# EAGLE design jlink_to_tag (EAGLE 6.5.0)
AUTHOR: Noah Klugman / Brad Campbell; REV: B; TITLE: JLink to Tag Connect
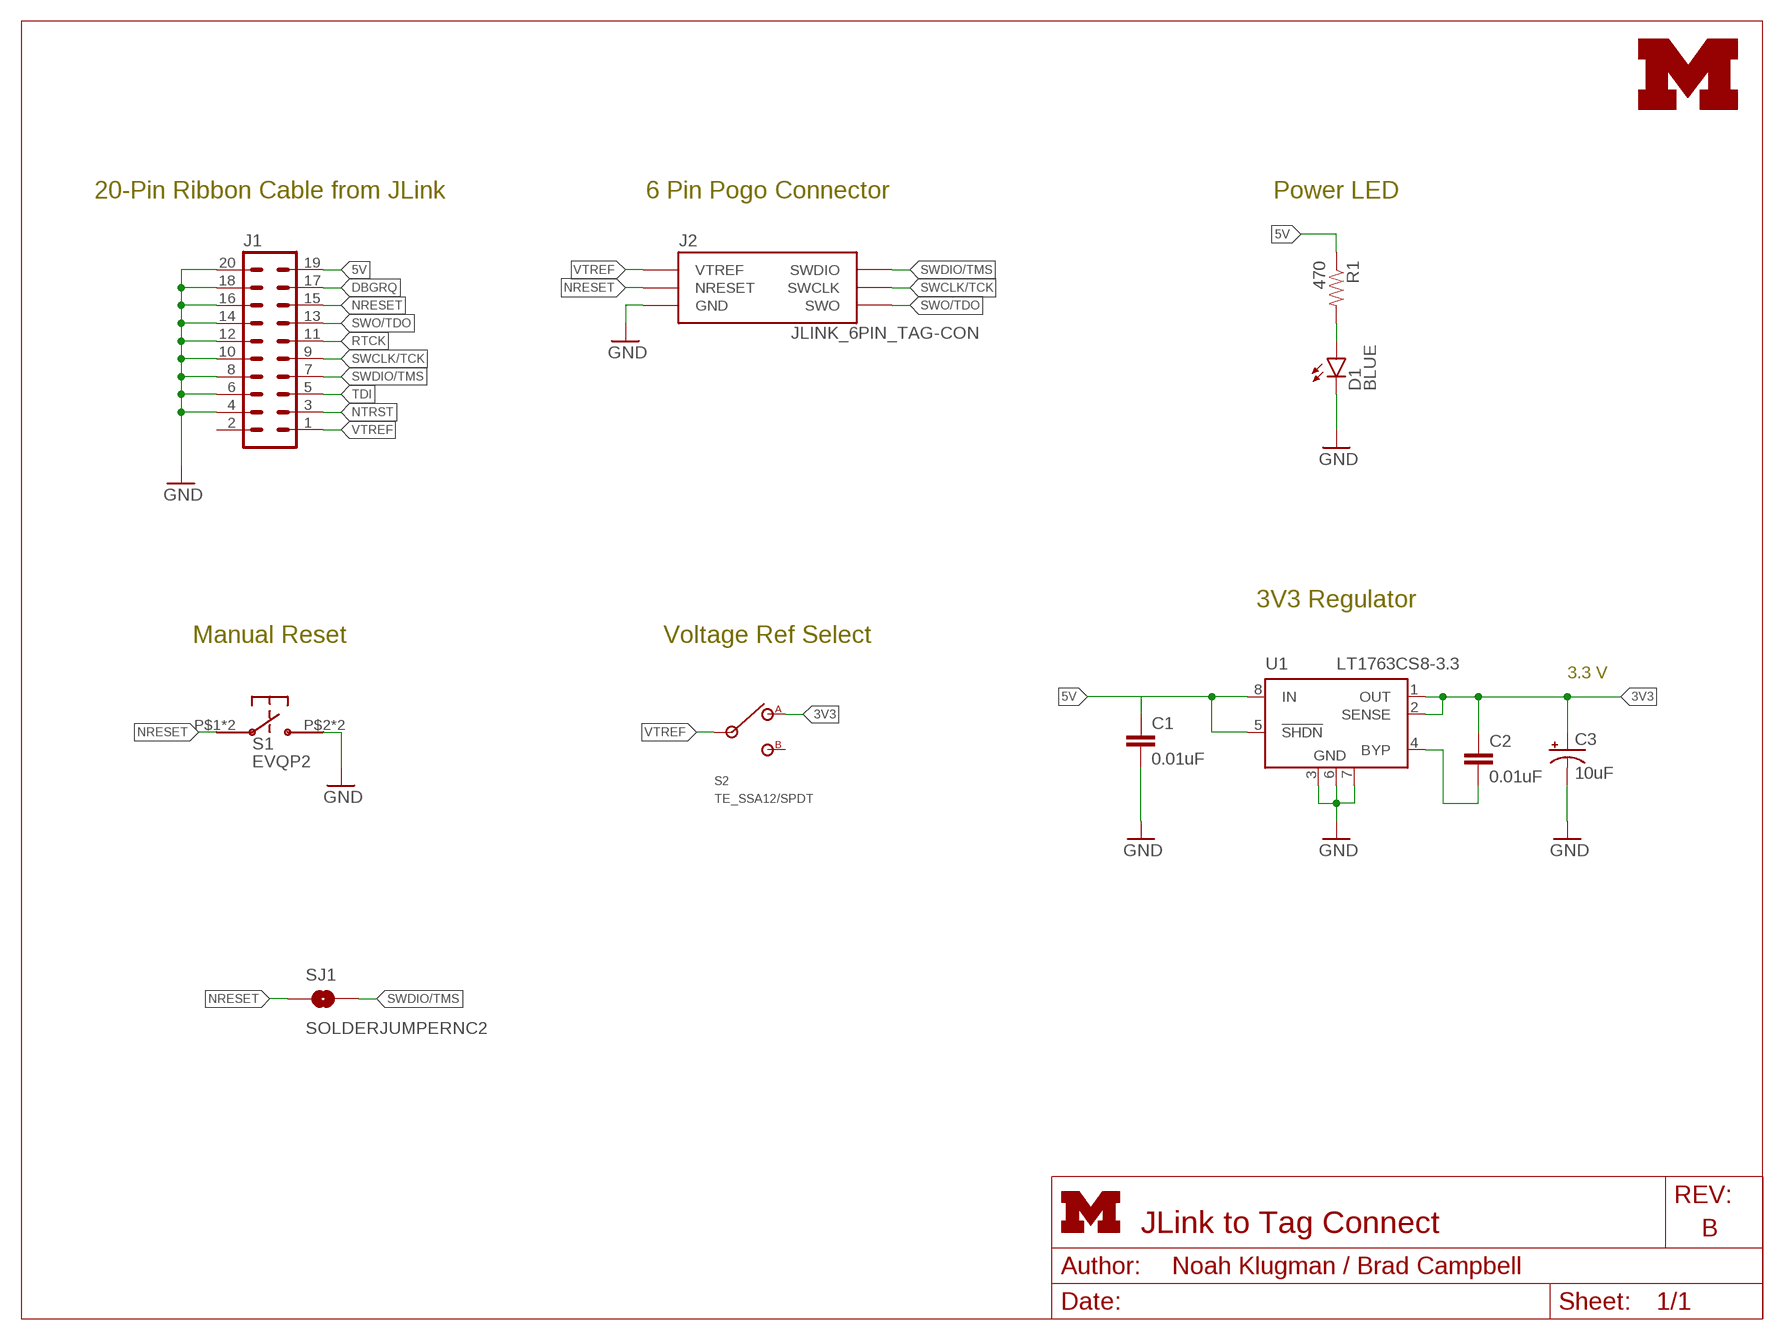
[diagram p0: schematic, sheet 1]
FRAME1 (LETTER_L): HEIGHT: 8.5in; WIDTH: 11in

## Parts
C1  0.01uF  C-EUC0603  [C0603]
C2  0.01uF  C-EUC0603  [C0603]
C3  10uF  CAP_POL1206  [EIA3216]
D1  BLUE  LED-BLUE0603  [LED-0603]
J1  ML20  [ML20]
J2  JLINK_6PIN_TAG-CON  [2X3_MALE_SHROUDED_0.100]
LOGO1  UMICH_SOLID_SMALL+  [UMICH_SOLID_100MIL]
R1  470  RESISTOR0603-RES  [0603-RES]
S1  EVQP2  [EVQP2]
S2  TE_SSA12/SPDT  [TE_SSA12/SPDT]
SJ1  SOLDERJUMPERNC2  [SJ_2S-NOTRACE]
U1  LT1763CS8-3.3  [SOIC8]

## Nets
3V3: C2.1 C3.A(+) S2.1(A) U1.1(OUT) U1.2(SENSE)
5V: C1.1 J1.19 R1.1 U1.5(!SHDN) U1.8(IN)
DBGRQ: J1.17
GND: C1.2 C3.C(-) D1.C J1.4 J1.6 J1.8 J1.10 J1.12 J1.14 J1.16 J1.18 J1.20 J2.5(GND) S1.P$2 S1.P$4 U1.3(GND) U1.6(GND) U1.7(GND)
N$3: D1.A R1.2
N$4: C2.2 U1.4(BYP)
NRESET: J1.15 J2.3(NRESET) S1.P$1 S1.P$3 SJ1.1
NTRST: J1.3
RTCK: J1.11
SWCLK/TCK: J1.9 J2.4(SWCLK)
SWDIO/TMS: J1.7 J2.2(SWDIO) SJ1.2
SWO/TDO: J1.13 J2.6(SWO)
TDI: J1.5
VTREF: J1.1 J2.1(VTREF) S2.IN
Unconnected: J1.2 S2.2(B)

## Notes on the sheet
- 20-Pin Ribbon Cable from JLink | 6 Pin Pogo Connector | Power LED
- 3V3 Regulator
- Manual Reset | Voltage Ref Select
- 3.3 V

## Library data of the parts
C1 C2 = resistor:C-EU: CAPACITOR, European symbol; DIGIKEY: 490-1512-1-ND
C3 = SparkFun-Passives:CAP_POL: Capacitor Polarized; DIGIKEY: 399-3684-1-ND
D1 = SparkFun-LED:LED-BLUE: Blue LEDs for production use; PROD_ID: DIO-08575
J1 = con-ml:ML20: HARTING; DIGIKEY: S9172-ND; OC_FARNELL: unknown; OC_NEWARK: unknown
J2 = headers:JLINK_6PIN_TAG-CON: This is a 6-pin Tag Connect header with the J-Link.; DIGIKEY: 3M15451-ND
LOGO1 = logos:UMICH_SOLID
R1 = SparkFun-Passives:RESISTOR: Resistor
S1 = switches:EVQP2: SWITCH TACTILE SPST-NO 0.02A 15V; DIGIKEY: P11084SCT-ND
S2 = switches:TE_SSA12/SPDT: SWITCH SLIDE SPDT 2POS SSA SER; DIGIKEY: 450-1602-ND
SJ1 = SparkFun-Passives:SOLDERJUMPER: Solder Jumper
U1 = linear-technology:LT1763CS8: 500mA, Low Noise, LDO Micropower Regulators Source: http://cds.linear.com/docs/Datasheet/1763ff.pdf; DIGIKEY: LT1763CS8-3.3#TRPBFCT-ND; MPN: LT1763CS8-3.3; OC_FARNELL: 1273617; OC_NEWARK: 57M6055

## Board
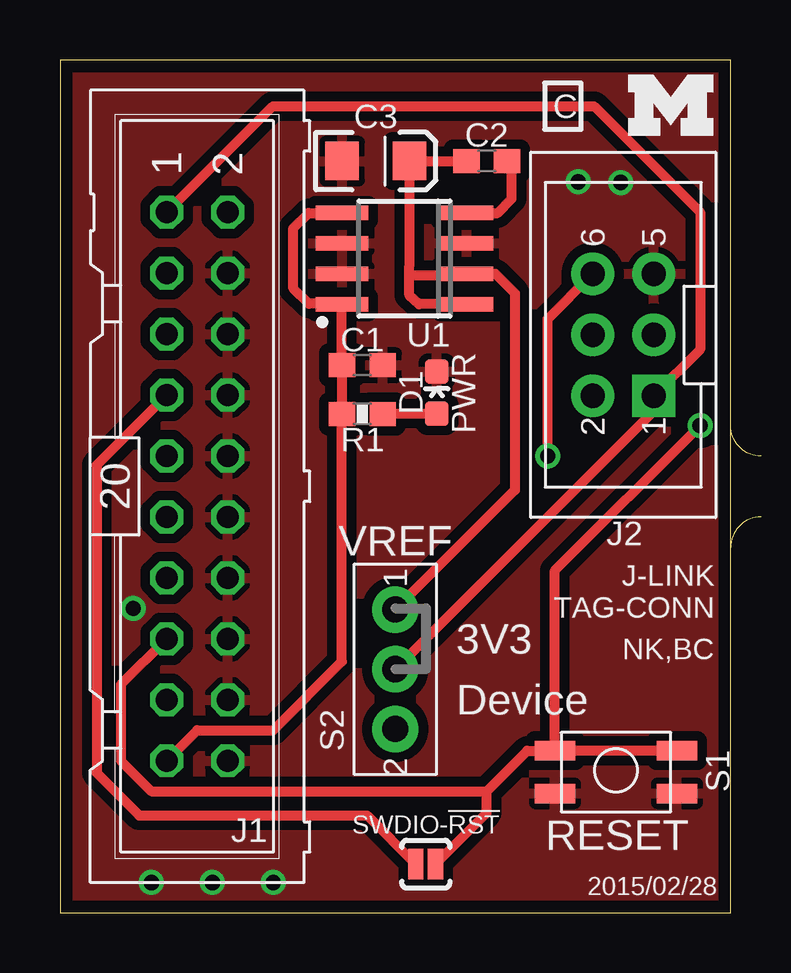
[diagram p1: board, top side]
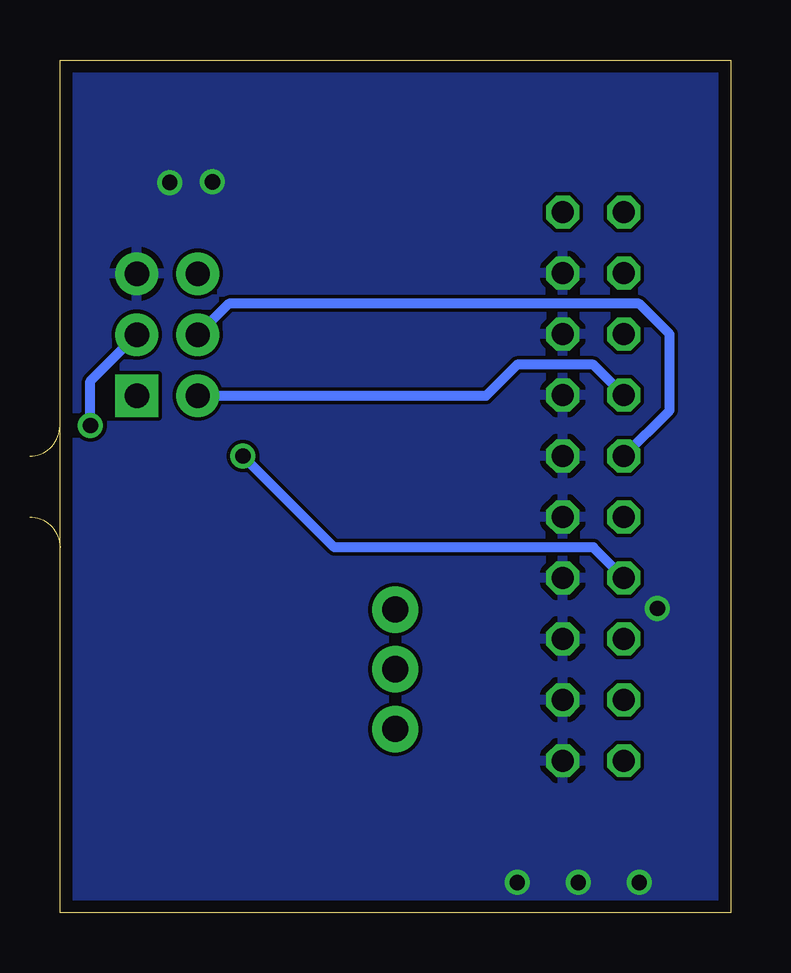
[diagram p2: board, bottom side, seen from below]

Size 27.94 x 35.56 mm. Coordinates in mm from the lower left corner, seen from the top.
Outline: 0,35.56 0,0 27.94,0 27.94,35.56 0,35.56
Copper layers (1*16): Top 0.0178mm / dielectric 59mil / Bottom 0.0178mm
Design rules "sunstone-2lyr_v1.0.0.3": minimum track width 6mil, minimum drill 14mil, track to track 6mil, track to pad 6mil, pad to pad 6mil, via to via 6mil, smd to smd 6mil, copper to edge 20mil, drill to drill 16mil, minimum pad ring 8mil, minimum via ring 8mil, stop-mask expansion 3mil, vias tented up to drill 0mil, thermal gap 10mil
Milling: 7 lines

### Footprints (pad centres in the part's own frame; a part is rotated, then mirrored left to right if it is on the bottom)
C0603 = smd 1.1 x 1: 1 -0.85,0; 2 0.85,0
EIA3216 = smd 1.4 x 1.6: A 1.4,0; C -1.4,0
LED-0603 = smd 1 x 1: A 0,-0.877; C 0,0.877
ML20 = drill 0.914 octagon: 1 -11.43,-1.27; 2 -11.43,1.27; 3 -8.89,-1.27; 4 -8.89,1.27; 5 -6.35,-1.27; 6 -6.35,1.27; 7 -3.81,-1.27; 8 -3.81,1.27; 9 -1.27,-1.27; 10 -1.27,1.27; 11 1.27,-1.27; 12 1.27,1.27; 13 3.81,-1.27; 14 3.81,1.27; 15 6.35,-1.27; 16 6.35,1.27; 17 8.89,-1.27; 18 8.89,1.27; 19 11.43,-1.27; 20 11.43,1.27
2X3_MALE_SHROUDED_0.100 = drill 1.016 pad 1.778 square: 1 -2.54,-1.27 | drill 1.016 pad 1.778: 2 -2.54,1.27; 3 0,-1.27; 4 0,1.27; 5 2.54,-1.27; 6 2.54,1.27
0603-RES = smd 1.1 x 1: 1 -0.85,0; 2 0.85,0
EVQP2 = smd 1.676 x 0.813: P$1 -2.54,-0.87; P$2 -2.54,0.908; P$3 2.54,-0.87; P$4 2.54,0.908
TE_SSA12/SPDT = drill 1.092 pad 1.93: 1 -2.489,0; 2 2.489,0; IN 0,0
SJ_2S-NOTRACE = smd 0.635 x 1.27: 1 -0.401,0; 2 0.413,0
SOIC8 = smd 0.6 x 2.2: 1 -1.905,-2.6; 2 -0.635,-2.6; 3 0.635,-2.6; 4 1.905,-2.6; 5 1.905,2.6; 6 0.635,2.6; 7 -0.635,2.6; 8 -1.905,2.6

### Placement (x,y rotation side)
C1  12.6,22.83 0 top
C2  17.78,31.34 0 top
C3  13.16,31.34 0 top
D1  15.7,21.69 0 top
J1  5.71,17.78 270 top
J2  23.47,24.1 90 top
LOGO1  23.67,32.41 0 top
R1  12.6,20.8 0 top
S1  23.16,5.89 180 top
S2  13.97,10.16 270 top
SJ1  15.24,2.03 180 top
U1  14.35,27.28 90 top

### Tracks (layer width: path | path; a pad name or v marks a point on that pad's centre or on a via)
3V3
  Top 0.406: U1.1 14.96,25.38 14.55,25.76 14.55,26.67 | 14.55,26.67 14.55,26.99 14.56,27 C3.A C2.1 | 14.55,26.67 14.63,26.59 16.93,26.59 U1.2 18.14,26.64 18.95,25.83 18.95,17.63 S2.1
5V
  Top 0.406: 11.76,29.22 U1.5 10.36,29.18 9.73,28.55 9.73,26.04 10.37,25.4 11.75,25.4 | C1.1 11.75,25.4 | 11.75,25.4 U1.8 | 11.77,22.84 C1.1 | C1.1 R1.1 11.75,10.48 8.89,7.62 5.71,7.62 J1.19
GND  (via drill 0.64)
  other vias: 3.81,1.27 6.35,1.27 8.89,1.27 21.59,30.48 23.37,30.45 3.05,12.7
  pour Top (isolate 0.406): -1.27,-1.27 29.21,-1.27 29.21,36.83 -1.27,36.83
  pour Bottom: -1.27,36.83 29.21,36.83 29.21,-1.27 -1.27,-1.27
N$3
  Top 0.406: 15.68,20.83 D1.A 13.46,20.82 R1.2
N$4
  Top 0.406: U1.4 18.24,29.18 18.82,29.77 18.82,31.15 C2.2
NRESET  (via drill 0.64)
  Top 0.406: J1.15 2.54,9.53 2.54,6.35 3.81,5.08 17.78,5.08 | S1.P$1 S1.P$3 | S1.P$3 20.62,14.28 v26.67,20.32 | 17.78,5.08 19.46,6.76 S1.P$3 | SJ1.1 17.78,4.17 17.78,5.08
  Bottom 0.406: v26.67,20.32 26.67,22.17 J2.3
SWCLK/TCK
  Bottom 0.406: J1.9 2.54,20.95 2.54,24.13 3.81,25.4 20.9,25.4 J2.4
SWDIO/TMS
  Top 0.406: J1.7 1.52,18.67 1.52,5.84 3.3,4.06 12.79,4.06 SJ1.2
  Bottom 0.406: J2.2 10.19,21.57 8.89,22.86 5.71,22.86 J1.7
SWO/TDO  (via drill 0.64)
  Top 0.406: v20.32,19.05 20.32,24.77 J2.6
  Bottom 0.406: J1.13 5.71,15.24 16.51,15.24 v20.32,19.05
VTREF
  Top 0.406: S2.IN 24.74,20.93 J2.1 26.67,23.5 26.67,29.21 22.25,33.63 8.87,33.63 J1.1

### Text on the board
tPlace: C | PWR | VREF | J-LINK / TAG-CONN | 3V3 | NK,BC | Device | RESET | SWDIO-!RST | 2015/02/28

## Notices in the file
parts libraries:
SparkFun-Passives: Licensing: Creative Commons ShareAlike 4.0 International - https://creativecommons.org/licenses/by-sa/4.0
